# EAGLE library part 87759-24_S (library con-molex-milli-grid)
HEADER
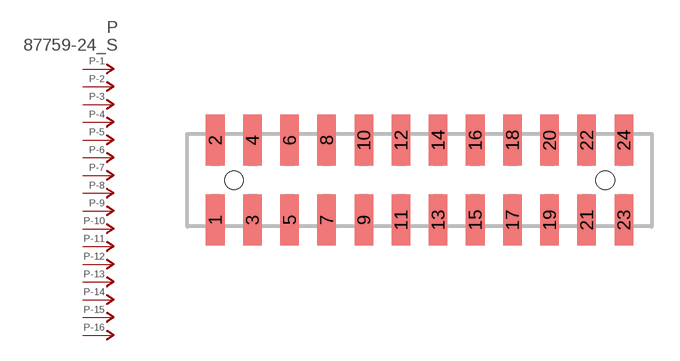
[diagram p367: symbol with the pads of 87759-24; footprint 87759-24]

Designator prefix P; gates -1=P-NV -2=P-N -3=P-N -4=P-N -5=P-N -6=P-N -7=P-N -8=P-N -9=P-N -10=P-N -11=P-N -12=P-N -13=P-N -14=P-N -15=P-N -16=P-N -17=P-N -18=P-N -19=P-N -20=P-N -21=P-N -22=P-N -23=P-N -24=P-N

## 87759-24_S  [87759-24]
1  -1:P  pas
2  -2:P  pas
3  -3:P  pas
4  -4:P  pas
5  -5:P  pas
6  -6:P  pas
7  -7:P  pas
8  -8:P  pas
9  -9:P  pas
10  -10:P  pas
11  -11:P  pas
12  -12:P  pas
13  -13:P  pas
14  -14:P  pas
15  -15:P  pas
16  -16:P  pas
17  -17:P  pas
18  -18:P  pas
19  -19:P  pas
20  -20:P  pas
21  -21:P  pas
22  -22:P  pas
23  -23:P  pas
24  -24:P  pas

## Footprint 87759-24 (pad centres in mm)
HEADER SMD Dual Row, Vertical
smd 1 x 2.75: 1 -11,-2.15; 2 -11,2.15; 3 -9,-2.15; 4 -9,2.15; 5 -7,-2.15; 6 -7,2.15; 7 -5,-2.15; 8 -5,2.15; 9 -3,-2.15; 10 -3,2.15; 11 -1,-2.15; 12 -1,2.15; 13 1,-2.15; 14 1,2.15; 15 3,-2.15; 16 3,2.15; 17 5,-2.15; 18 5,2.15; 19 7,-2.15; 20 7,2.15; 21 9,-2.15; 22 9,2.15; 23 11,-2.15; 24 11,2.15
hole 1 at -10,0
hole 1 at 10,0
